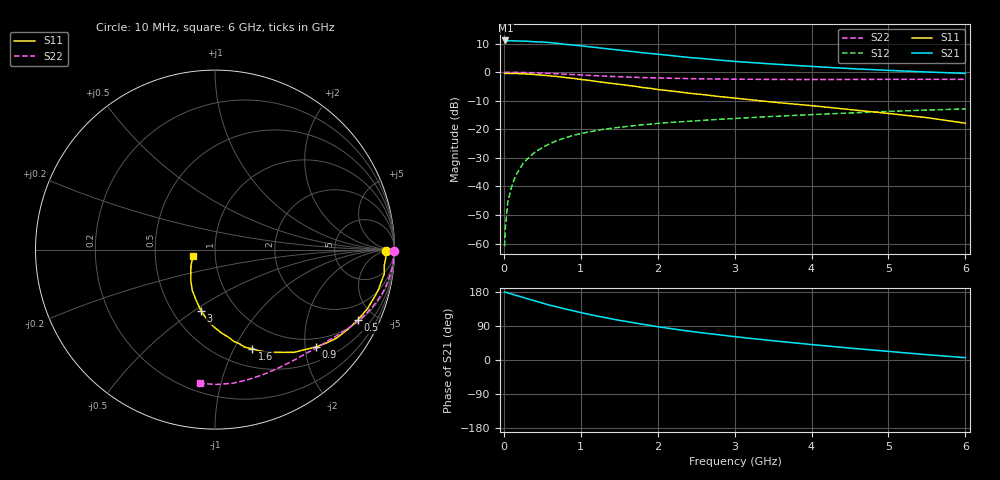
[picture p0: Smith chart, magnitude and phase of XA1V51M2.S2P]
! SIEMENS Discrete & RF Semiconductors
! BFY180
! Si NPN RF Bipolar Junction Transistor in MICRO-X
! VCE = 1.5 V  IC = 1.2 mA
! Common Emitter S-Parameters:  May  1997
# GHz  S  MA  R  50
!  f  S11  S21  S12  S22
! GHz  MAG  ANG  MAG  ANG  MAG  ANG  MAG  ANG
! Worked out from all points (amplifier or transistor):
!   36 points, 10 MHz to 6 GHz, reference 50 ohm
!   highest |S21| = 11.1 dB at 20 MHz (marker M1)
!   |S21| within 3 dB of that: start of sweep to 1.371 GHz
!   unconditionally stable (mu >= 1): 3.125 GHz to end of sweep
!   at 250 MHz: K = 0.11, MSG = 21.4 dB, |S12| = -31.9 dB
!   at 1.4 GHz: K = 0.60, MSG = 13.8 dB, |S12| = -19.7 dB
!   at 6 GHz: K = 1.09, MAG = 4.4 dB, |S12| = -12.9 dB
!   S11 on the Smith chart (normalised r, x): 10 MHz: 42, -6; 500 MHz: 1.08, -3.99; 900 MHz: 0.80, -2.22; 1.6 GHz: 0.70, -1.18; 3 GHz: 0.69, -0.54; 6 GHz: 0.78, -0.06
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0.01  0.9546 -0.4  3.555 179.6  0.0009 97.8  0.9958 -0.3
0.02  0.9474 -1.1  3.597 178.7  0.0019 87.5  0.998 -0.6
0.05  0.953 -2.6  3.534 177.2  0.0052 84.6  0.9972 -1.4
0.1  0.9469 -5.4  3.564 174.2  0.0098 87.2  0.9947 -3.0
0.15  0.9528 -8.1  3.535 171.2  0.0152 85.3  0.9959 -4.4
0.25  0.9374 -13.7  3.5 165.2  0.0253 80.8  0.9895 -7.4
0.3  0.9296 -15.9  3.492 162.0  0.0298 79.6  0.984 -8.7
0.5  0.8864 -26.4  3.377 150.3  0.0479 72.3  0.9657 -14.2
0.6  0.8633 -30.9  3.303 144.3  0.0563 69.4  0.9513 -16.8
0.9  0.78 -44.1  2.991 129.9  0.0783 60.1  0.9103 -23.7
1.1  0.7225 -52.4  2.797 120.8  0.0894 55.6  0.8819 -27.7
1.2  0.6909 -56.0  2.709 116.5  0.0952 53.5  0.8694 -29.7
1.4  0.638 -63.3  2.521 108.5  0.1041 49.8  0.8442 -33.2
1.6  0.59 -69.4  2.349 101.5  0.1123 46.8  0.8239 -36.4
2  0.4976 -80.8  2.068 87.7  0.1271 41.8  0.7943 -42.4
2.2  0.4664 -85.5  1.94 82.0  0.1331 39.4  0.783 -45.3
2.6  0.4037 -94.7  1.725 71.2  0.144 35.8  0.765 -50.5
3  0.3523 -102.6  1.546 61.6  0.1549 32.4  0.755 -55.7
3.5  0.2992 -110.8  1.389 50.8  0.1684 28.8  0.7481 -62.1
4.5  0.2217 -127.3  1.158 31.4  0.1934 21.2  0.7475 -75.2
5.5  0.1602 -146.7  1.01 14.0  0.2173 13.5  0.7514 -89.2
6  0.128 -162.8  0.954 6.2  0.2277 9.3  0.7502 -96.3
